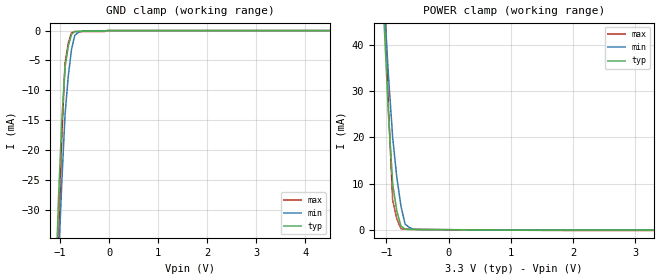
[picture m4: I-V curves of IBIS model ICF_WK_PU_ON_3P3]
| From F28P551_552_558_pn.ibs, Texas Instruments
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|   Model Cell ICF_WK_PU_ON_3P3
|ICF_WK_PU_ON_3P3
[Model]   ICF_WK_PU_ON_3P3
Model_type   Input
Polarity   Non-Inverting
Vinl =  0.8
Vinh =  2
C_comp   0.705929p   0.524756p   0.819798p
[Model Spec]
Vinl   0.8   0.8   0.8
Vinh   2   2   2
[Temperature Range]   25   155   -40
[Voltage Range]   3.3   2.97   3.63
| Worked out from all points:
|   GND clamp passes 1 mA (typ) near -0.78 V on its own axis
|   POWER clamp passes 1 mA (typ) near -0.77 V on its own axis
| Nom Voltages:
|   BIASFET=3.3, VDD=1.2, VDDS=3.3, VSS=0
| Min Voltages:
|   BIASFET=2.97, VDD=1.08, VDDS=2.97, VSS=0
| Max Voltages:
|   BIASFET=3.63, VDD=1.32, VDDS=3.63, VSS=0
[POWER_clamp]
|   voltage   I(typ)   I(min)   I(max)
-3.3V     1.081A     1.025A     1.649A
-1.033V   43.64mA    48.41mA    54.09mA
-966.7mV  24.74mA    33.21mA    26.16mA
-900mV    9.881mA    19.98mA    6.383mA
-833.3mV  4.056mA    11.34mA    2.316mA
-766.7mV  796.5uA    5.088mA    220.1uA
-700mV    101.7uA    1.216mA    96.03uA
-633.3mV  72.36uA    499uA      85.21uA
-566.7mV  53.97uA    105.2uA    75.1uA
3.3V      -108.6uA   -51.41uA   -173.9uA
[GND_clamp]
|   voltage   I(typ)   I(min)   I(max)
-3.3V     -921.9mA   -819.9mA   -1.722A
-1.1V     -45.05mA   -53.7mA    -60.96mA
-1.033V   -28.29mA   -38.88mA   -36.6mA
-966.7mV  -15.33mA   -25.71mA   -18.14mA
-900mV    -6.156mA   -14.2mA    -5.575mA
-833.3mV  -2.606mA   -7.595mA   -2.143mA
-766.7mV  -601.1uA   -3.123mA   -345uA
-700mV    -141.8uA   -786.5uA   -179.4uA
-566.7mV  -109.9uA   -110.7uA   -175.2uA
-500mV    -109.1uA   -59.75uA   -175.1uA
-33.33mV  0A         0A         0A
6.6V      0A         0A         0A
